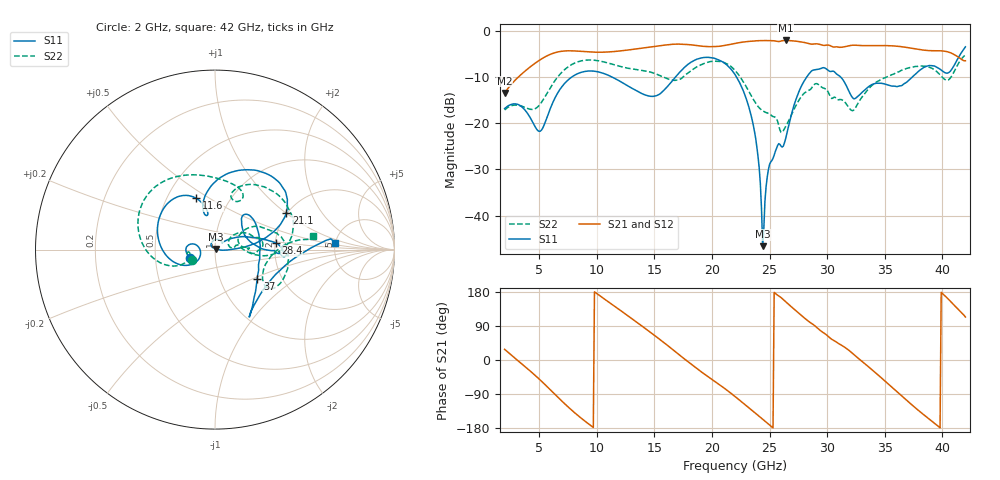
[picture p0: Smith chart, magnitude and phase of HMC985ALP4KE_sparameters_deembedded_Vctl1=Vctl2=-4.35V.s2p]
!s2p File: Measurements: S11, S21, S12, S22
# GHz S dB R 50.0
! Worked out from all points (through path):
!   401 points, 2 GHz to 42 GHz, reference 50 ohm
!   highest |S21| = -2.07 dB at 26.4 GHz (marker M1); lowest = -13.4 dB at 2 GHz (marker M2)
!   lowest |S11| = -46.6 dB at 24.4 GHz (marker M3), VSWR 1.01, Z = 50.4 + j0.286 ohm
!   |S11| at or under -10 dB: start of sweep to 7.824 GHz; 22.13 GHz to 28.22 GHz (6.089 GHz wide, 24.2 % of centre); 31.18 GHz to 37.38 GHz (6.208 GHz wide, 18.1 % of centre)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
!   |S22| runs from -22.0 to -5.2 dB; largest |S21 - S12| = 0.00069
!   S11 on the Smith chart (normalised r, x): 2 GHz: 0.76, -0.07; 11.6 GHz: 0.70, +0.44; 21.1 GHz: 1.98, +1.01; 28.4 GHz: 2.01, +0.17; 37 GHz: 1.50, -0.53; 42 GHz: 5.00, +0.70
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2  -16.81 -161.8  -13.44 28.2  -13.45 28.2  -17.11 -155.6
3.3  -16.10 173.3  -9.74 -5.3  -9.74 -5.3  -16.14 -173.4
5  -21.75 -173.6  -6.39 -50.2  -6.39 -50.2  -16.11 -160.3
6.3  -14.88 -150.8  -4.77 -88.5  -4.77 -88.5  -11.01 -162.0
8.7  -8.93 150.1  -4.45 -154.8  -4.45 -154.8  -6.46 151.0
11.6  -10.34 110.1  -4.45 140.7  -4.45 140.7  -7.39 103.1
13.6  -13.17 101.4  -3.84 96.8  -3.85 96.8  -8.44 75.3
15.4  -13.77 106.4  -3.24 55.9  -3.24 55.9  -9.57 62.0
17.9  -7.27 79.8  -2.95 -4.2  -2.95 -4.2  -9.14 72.0
21.1  -7.01 27.2  -3.15 -75.0  -3.15 -75.0  -6.90 15.5
22  -9.44 16.7  -2.71 -96.3  -2.71 -96.3  -8.53 0.1
23.6  -20.56 0.7  -2.19 -136.1  -2.18 -136.0  -14.86 -4.0
24.4  -46.61 37.5  -2.09 -156.2  -2.09 -156.2  -17.31 7.8
25  -28.91 129.3  -2.11 -171.5  -2.12 -171.5  -17.97 11.6
26.4  -23.30 41.6  -2.07 153.7  -2.07 153.7  -20.71 33.4
28.4  -9.38 6.3  -2.73 101.7  -2.74 101.7  -12.88 17.8
28.7  -8.58 1.3  -2.87 95.5  -2.88 95.5  -12.18 15.9
32.5  -14.51 33.5  -3.10 9.6  -3.10 9.6  -16.46 28.7
35.4  -11.77 18.3  -3.20 -65.9  -3.20 -65.9  -9.74 19.0
37  -10.88 -34.5  -3.62 -109.1  -3.62 -109.0  -8.06 4.3
39.8  -8.28 -56.7  -4.31 -178.9  -4.31 -178.9  -9.49 -35.2
42  -3.45 3.3  -6.46 113.4  -6.47 113.4  -5.20 7.9
